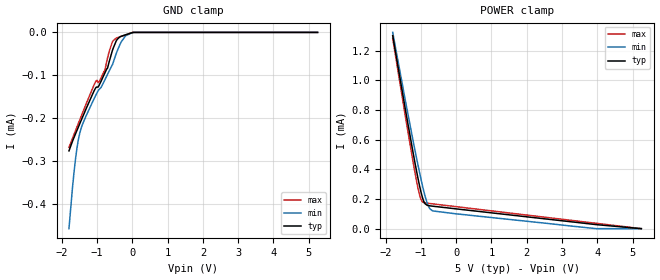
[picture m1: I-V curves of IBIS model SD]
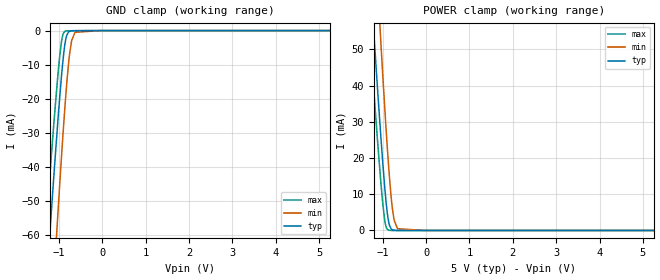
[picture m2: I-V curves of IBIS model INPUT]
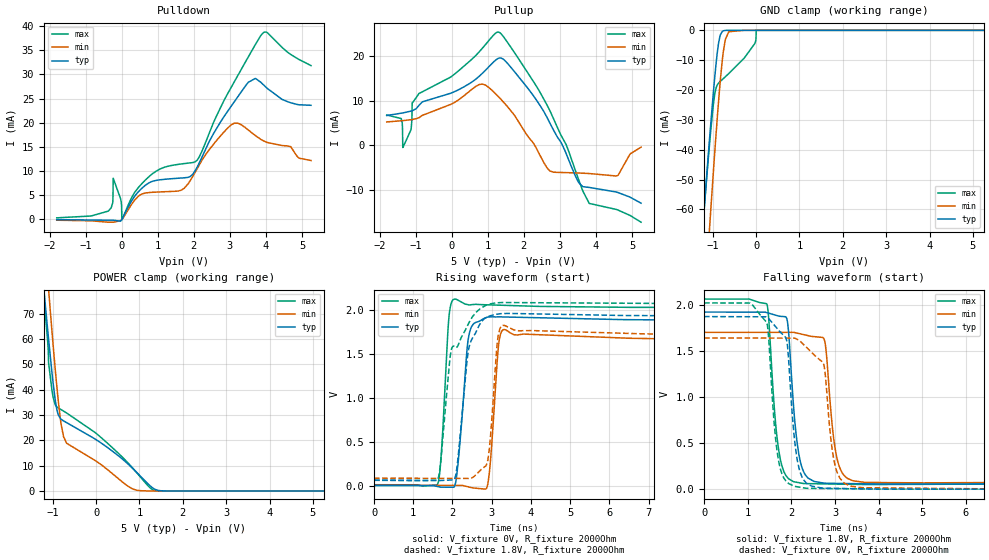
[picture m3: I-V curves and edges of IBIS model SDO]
|Texas Instruments Incorporated
|  5 GHz Ultra Wideband Digital Variable Gain Amplifier
| Marketing part#   Digital Voltage Range   Package-type   #pins
|  LMH6401   1.7V to 1.9V   QFN   16
[IBIS Ver]   4.1
[File name]   lmh6401.ibs
[File Rev]   1.0
[Date]   04/14/2015
[Source]
| Texas Instruments Incorporated.
| 12500 TI Blvd
| Dallas, TX -75243
[Notes]   Revision History:
| Rev 1.0: 04/14/2015
| - Initial version of the model
| - Model generated from simulations in TISPICE
| - C_comp although listed in numerical order of value are
|   obtained from varying PVT conditions. For PVT conditions for
|   each specific value refer the buffer description under
|   respective [Model]. IBIS model user is responsible for using
|   appropriate C_comp to simulate for Signal Integrity.
| - Warnings regarding combined Non-monotonicity of various models have been
|   reviewd and considered minor and can be ignored.
[Disclaimer]
| This model is designed as an aid for customers of Texas Instruments.
| TI and its licensors and suppliers make no warranties, either expressed
| or implied, with respect to this  model, including the warranties of
| merchantability or fitness for a particular purpose. The model is
| provided solely on an "as is" basis. The entire risk as to its quality
| and performance is with the customer.
[Copyright]
 (C) Copyright 2015 Texas Instruments Incorporated.All rights reserved.
|   Device
[Component]  LMH6401
[Manufacturer]   TI
[Package]  |QFN   16
|   typ   min   max
R_pkg   0.067   0.027   0.083
L_pkg   0.937nH   0.593nH   1.143nH
C_pkg   0.144pF   0.126pF   0.200pF
[Pin]  signal_name   model_name   R_pin   L_pin   C_pin
1   SDI   INPUT   NA   NA   NA
2   INM   NC   NA   NA   NA
3   INP   NC   NA   NA   NA
4   SDO   SDO   NA   NA   NA
5   VEE   GND   NA   NA   NA
6   PD   SD   NA   NA   NA
7   VOCM   NC   NA   NA   NA
8   VCC   POWER   NA   NA   NA
9   GND   GND   NA   NA   NA
10   OUTM   NC   NA   NA   NA
11   OUTP   NC   NA   NA   NA
12   GND   GND   NA   NA   NA
13   VCC   POWER   NA   NA   NA
14   CLK   INPUT   NA   NA   NA
15   CSNB   INPUT   NA   NA   NA
16   VEE   GND   NA   NA   NA
| Models and submodels in the file (3): SD (Input), INPUT (Input), SDO (I/O)
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|   Model
[Model]   SD
Model_type   Input
Vinl = 0.54
Vinh = 1.26
|   typ   min   max
C_comp   0.343pF   0.325pF   0.368pF
[Voltage Range]   5   4   5.25
[Temperature Range]   27   125   -40
[Power Clamp Reference]   5   4   5.25
[GND Clamp Reference]   0   0   0
[GND Clamp]
|   Voltage   I(typ)   I(min)   I(max)
-1.8V     -276.2uA   -457.4uA   -268.2uA
-1.701V   -253.9uA   -363.2uA   -247.4uA
-1.617V   -237.1uA   -296.9uA   -229.6uA
-1.539V   -221.8uA   -252.6uA   -213.4uA
-1.455V   -205.3uA   -223.3uA   -195.8uA
-1.046V   -129.9uA   -147.6uA   -115.3uA
-954mV    -124.8uA   -133.9uA   -116.5uA
-791.9mV  -96.31uA   -112.3uA   -91.97uA
-559.2mV  -40.05uA   -73.62uA   -20.94uA
-432.3mV  -16.37uA   -43.39uA   -12.46uA
-192.6mV  -5.592uA   -7.87uA    -5.643uA
5.25V     0A         0A         0A
[POWER Clamp]
|   Voltage   I(typ)   I(min)   I(max)
-1.8V     1.302mA    1.325mA    1.284mA
-1.455V   823.5uA    881.5uA    777.6uA
-1.229V   521.7uA    601.6uA    459.2uA
-1.137V   405.2uA    492uA      338.5uA
-1.039V   289.1uA    378.7uA    227.9uA
-996.3mV  245.2uA    332.3uA    196.4uA
-897.6mV  174uA      233.1uA    174.8uA
-806mV    156.8uA    161.5uA    171.4uA
-749.6mV  154.2uA    134.8uA    169.7uA
-672mV    151.7uA    119.9uA    167.5uA
3.974V    27.18uA    0A         36.04uA
5.25V     0A         0A         0A
|   Model
[Model]   INPUT
Model_type   Input
Vinl = 0.54
Vinh = 1.26
|   typ   min   max
C_comp   0.343pF   0.325pF   0.368pF
[Voltage Range]   5   4   5.25
[Temperature Range]   27   125   -40
[Power Clamp Reference]   5   4   5.25
[GND Clamp Reference]   0   0   0
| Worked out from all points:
|   GND clamp passes 1 mA (typ) near -0.80 V on its own axis
|   POWER clamp passes 1 mA (typ) near -0.83 V on its own axis
[GND Clamp]
|   Voltage   I(typ)   I(min)   I(max)
-1.8V     -172.8mA   -226.5mA   -145.4mA
-1.384V   -92.32mA   -132mA     -72.25mA
-1.173V   -52.69mA   -85.25mA   -36.26mA
-1.088V   -37.45mA   -67.09mA   -22.59mA
-1.024V   -26.5mA    -53.82mA   -13.06mA
-939.9mV  -13.16mA   -36.82mA   -3.1mA
-862.3mV  -3.979mA   -22.46mA   -236.3uA
-820mV    -1.386mA   -15.48mA   -91.34uA
-756.6mV  -226.1uA   -7.029mA   -58.04uA
-707.3mV  -89.29uA   -2.907mA   -40.23uA
-629.7mV  -43.71uA   -506.1uA   -18.11uA
5.25V     0A         0A         0A
[POWER Clamp]
|   Voltage   I(typ)   I(min)   I(max)
-1.8V     168.6mA    222.4mA    141.7mA
-1.398V   90.89mA    130mA      71.45mA
-1.187V   51.29mA    82.76mA    35.68mA
-1.109V   37.33mA    65.96mA    23.21mA
-1.039V   25.2mA     51.09mA    12.67mA
-954mV    12.05mA    34.08mA    2.879mA
-883.5mV  3.897mA    21.1mA     233.7uA
-841.2mV  1.335mA    14.22mA    41.89uA
-777.8mV  194.5uA    6.122mA    2.436uA
-735.5mV  50.12uA    2.799mA    500.4nA
-657.9mV  3.336uA    491.6uA    161.5nA
5.25V     0A         0A         0A
|   Model
[Model]   SDO
Model_type   I/O
Polarity   Non-Inverting
Enable   Active-Low
Vinl = 0.54
Vinh = 1.26
Vmeas = 0.9
Vref = 0
Cref = 1pF
Rref = 100000
|   typ   min   max
C_comp   0.489pF   0.469pF   0.517pF
[Voltage Range]   5   4   5.25
[Temperature Range]   27   125   -40
[Pullup Reference]   5   4   5.25
[Pulldown Reference]   0   0   0
[Power Clamp Reference]   5   4   5.25
[GND Clamp Reference]   0   0   0
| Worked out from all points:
|   slope of the pulldown table from 0 to 0.75 V, typ, clamps not added: 99.1 ohm
|   GND clamp passes 1 mA (typ) near -0.80 V on its own axis
|   falling waveform, V_fixture 1.8V, R_fixture 2000Ohm: 20-80 % time 193ps typ, 196ps min, 192ps max; typ from 1.92 V to 0.067 V
|   rising waveform, V_fixture 0V, R_fixture 2000Ohm: 20-80 % time 194ps typ, 148ps min, 144ps max; typ from 0.004 V to 1.87 V
|   rising waveform, V_fixture 1.8V, R_fixture 2000Ohm: 20-80 % time 245ps typ, 161ps min, 466ps max; typ from 0.067 V to 1.92 V
|   falling waveform, V_fixture 0V, R_fixture 2000Ohm: 20-80 % time 195ps typ, 211ps min, 191ps max; typ from 1.87 V to 0.004 V
[Pulldown]
|   Voltage   I(typ)   I(min)   I(max)
-1.8V     -69.16uA   -183.9uA   304.9uA
-375.9mV  -180.5uA   -593.8uA   1.694mA
-249mV    -178uA     -590.4uA   3.386mA
-234.9mV  -177.5uA   -592.5uA   8.496mA
-30.45mV  -389.8uA   -296uA     4.29mA
4.8mV     7.466uA    -21.56uA   -127.2uA
836.7mV   7.825mA    5.586mA    9.335mA
1.647V    8.548mA    6.021mA    11.46mA
2.085V    10.69mA    10.36mA    12.19mA
3.128V    24.39mA    19.91mA    28.54mA
3.946V    27.74mA    16.19mA    38.75mA
5.25V     23.6mA     12.17mA    31.82mA
[GND Clamp]
|   Voltage   I(typ)   I(min)   I(max)
-1.8V     -180.7mA   -235mA     -175.4mA
-1.384V   -96.58mA   -137mA     -95.06mA
-1.194V   -59.18mA   -93.28mA   -59.44mA
-1.088V   -39.17mA   -69.67mA   -40.68mA
-1.046V   -31.47mA   -60.45mA   -33.7mA
-946.9mV  -14.82mA   -39.69mA   -20.96mA
-862.3mV  -4.127mA   -23.35mA   -17.66mA
-770.7mV  -281.1uA   -8.986mA   -16.38mA
-629.7mV  -1.381uA   -473.1uA   -14.49mA
-30.45mV  0A         -66.55pA   -4.457mA
4.8mV     0A         0A         -7.9uA
5.25V     0A         0A         0A
[Pullup]
|   Voltage   I(typ)   I(min)   I(max)
-1.8V     6.653mA    5.22mA     6.768mA
-1.398V   7.17mA     5.475mA    5.966mA
-1.37V    7.21mA     5.495mA    4.943mA
-1.356V   7.231mA    5.506mA    -490.5uA
-1.095V   7.718mA    5.755mA    9.476mA
-904.6mV  8.93mA     6.167mA    11.58mA
759.1mV   15.38mA    13.54mA    20.83mA
1.316V    19.47mA    10.68mA    25.22mA
2.733V    4.806mA    -5.763mA   7.552mA
3.812V    -9.4mA     -6.3mA     -12.94mA
4.594V    -10.5mA    -6.767mA   -14.41mA
5.25V     -12.92mA   -409.9uA   -17.16mA
[POWER Clamp]
|   Voltage   I(typ)   I(min)   I(max)
-1.8V     196.2mA    241.2mA    186.8mA
-1.398V   116.8mA    147.4mA    111.5mA
-1.173V   73.89mA    96.41mA    69.87mA
-1.116V   63.63mA    84.05mA    59.13mA
-1.095V   59.87mA    79.48mA    50.54mA
-989.2mV  42.41mA    57.37mA    36.89mA
-904.6mV  32.21mA    41.21mA    33.23mA
-806mV    28.3mA     26.32mA    32.09mA
-679.1mV  26.96mA    18.82mA    30.77mA
759.1mV   10.27mA    1.604mA    10.62mA
1.394V    393.4uA    543.6nA    73.66uA
5.25V     0A         0A         0A
[Ramp]
R_load = 2000
|   typ   min   max
dV/dt_r   1.12145/1.94105e-10   0.980668/1.47882e-10   1.20462/1.44202e-10
dV/dt_f   1.11329/1.93271e-10   0.968616/1.95181e-10   1.19968/1.91888e-10
[Falling Waveform]
V_fixture = 1.8V
V_fixture_min = 1.8V
V_fixture_max = 1.8V
R_fixture = 2000Ohm
C_fixture = 0F
|   Time   V(typ)   V(min)   V(max)
0s        1.922V     1.702V     2.063V
1.433ns   1.917V     1.703V     2.013V
1.663ns   1.885V     1.703V     602.3mV
1.873ns   1.872V     1.703V     153.8mV
2.109ns   597mV      1.697V     79.33mV
2.281ns   192.2mV    1.678V     64.51mV
2.742ns   69.46mV    1.638V     60.69mV
3.066ns   65.54mV    297.9mV    58.29mV
3.663ns   61.68mV    78.12mV    53.87mV
50ns      66.58mV    88.14mV    63.66mV
[Rising Waveform]
V_fixture = 0V
V_fixture_min = 0V
V_fixture_max = 0V
R_fixture = 2000Ohm
C_fixture = 0F
|   Time   V(typ)   V(min)   V(max)
0s        4.026mV    6.829mV    13.48mV
1.611ns   -5.715mV   6.456mV    10.68mV
1.711ns   -14.42mV   6.432mV    341.8mV
1.902ns   -14.55mV   6.388mV    1.879V
2.051ns   -5.481mV   6.353mV    2.119V
2.417ns   1.703V     -12.06mV   2.054V
2.972ns   1.918V     305.5mV    2.053V
3.174ns   1.917V     1.593V     2.05V
3.318ns   1.916V     1.774V     2.048V
50ns      1.873V     1.641V     2.021V
[Rising Waveform]
V_fixture = 1.8V
V_fixture_min = 1.8V
V_fixture_max = 1.8V
R_fixture = 2000Ohm
C_fixture = 0F
|   Time   V(typ)   V(min)   V(max)
0s        66.56mV    88.11mV    63.78mV
1.611ns   61.16mV    85.8mV     65.54mV
1.687ns   61.11mV    85.69mV    219.8mV
1.945ns   67.03mV    85.32mV    1.478V
2.038ns   69.17mV    85.18mV    1.584V
2.417ns   1.561V     84.64mV    1.848V
2.873ns   1.912V     246.3mV    2.052V
3.097ns   1.946V     1.378V     2.076V
3.284ns   1.954V     1.821V     2.08V
50ns      1.922V     1.702V     2.063V
[Falling Waveform]
|Gnd
V_fixture = 0V
V_fixture_min = 0V
V_fixture_max = 0V
R_fixture = 2000Ohm
C_fixture = 0F
|   Time   V(typ)   V(min)   V(max)
0s        1.873V     1.641V     2.021V
1.433ns   1.866V     1.64V      1.811V
1.663ns   1.751V     1.64V      453.8mV
1.873ns   1.647V     1.64V      94.07mV
2.109ns   400.4mV    1.633V     31.24mV
2.322ns   81.05mV    1.551V     14.13mV
2.742ns   14.97mV    1.354V     10.6mV
3.05ns    11.5mV     184.5mV    9.128mV
3.565ns   7.813mV    21.78mV    6.67mV
50ns      4.016mV    6.826mV    13.24mV
